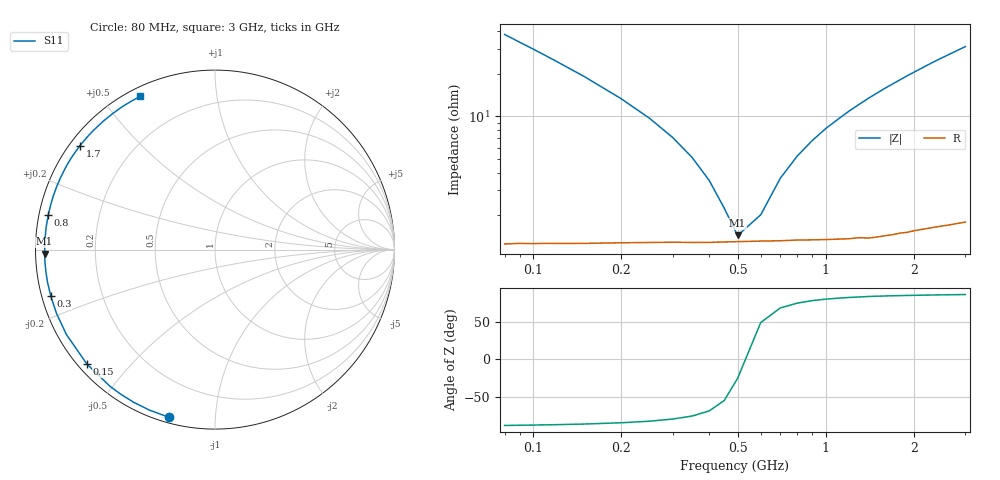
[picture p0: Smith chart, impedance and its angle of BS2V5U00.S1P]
! SIEMENS Small Signal Semiconductors
! BB640
! Si Tuning Diode in SOD323
! VR = 2.5 V
! S-Parameters:  July  1993
# GHz  S  MA  R  50
!  f  S11
! GHz  MAG  ANG
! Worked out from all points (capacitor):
!   33 points, 80 MHz to 3 GHz, reference 50 ohm
!   read as one part to ground: C = 51.1 pF near 80 MHz
!   lowest |Z| = 1.43 ohm at 500 MHz (marker M1)
!   series resonance near 528.6 MHz, so ESL is about 1.8 nH
!   S11 on the Smith chart (normalised r, x): 80 MHz: 0.02, -0.76; 150 MHz: 0.03, -0.38; 300 MHz: 0.03, -0.14; 800 MHz: 0.03, +0.10; 1.7 GHz: 0.03, +0.34; 3 GHz: 0.04, +0.62
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0.08  0.9689 -105.4
0.09  0.9659 -112.2
0.1  0.9638 -118.0
0.11  0.9618 -123.1
0.12  0.9603 -127.6
0.15  0.957 -138.2
0.2  0.9536 -150.2
0.25  0.9519 -158.2
0.3  0.9509 -164.1
0.35  0.9506 -168.7
0.4  0.9503 -172.5
0.45  0.9498 -175.8
0.5  0.9495 -178.6
0.6  0.9491 176.5
0.7  0.949 172.2
0.8  0.9487 168.4
0.9  0.9489 164.9
1  0.9491 161.6
1.2  0.9494 155.6
1.4  0.95 150.0
1.6  0.9494 144.8
1.7  0.9492 142.4
1.9  0.9489 137.6
2  0.9484 135.4
2.2  0.9484 131.0
2.4  0.9485 126.9
2.8  0.9494 119.5
3  0.95 116.0
